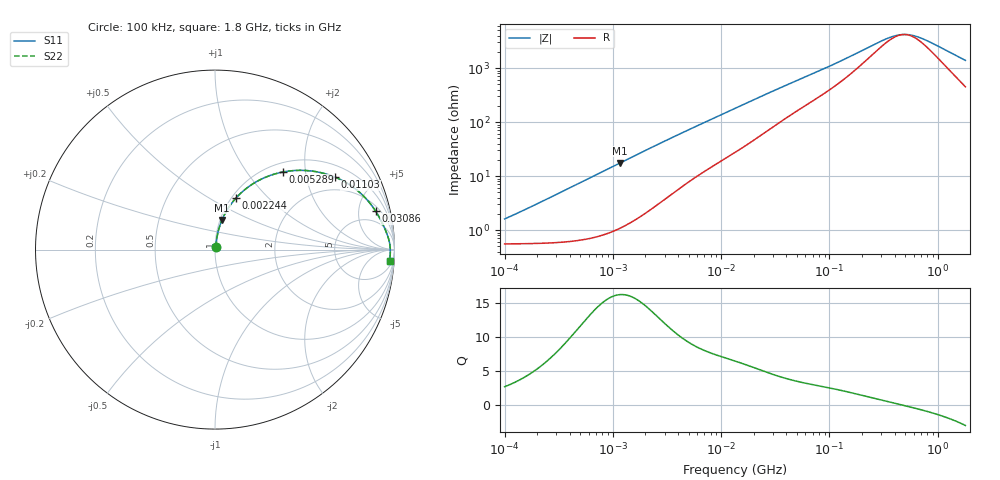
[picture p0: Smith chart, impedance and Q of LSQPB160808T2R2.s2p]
! LSQPB160808T2R2  S-PARAMETER MODEL  ( General Type )
! Model Generated by TAIYO YUDEN Corporation (http://www.ty-top.com)
! Version 4.0
! TAIYO YUDEN Control No. 100810NF18SB-HKC
! Copyright(c) 2007 TAIYO YUDEN CO.,LTD. All Rights Reserved.
! Product Description (link to TY-COMPAS)
! https://ds.yuden.co.jp/TYCOMPAS/or/detail?pn=LSQPB160808T2R2M&u=M
! Products Name : Inductors
! Characteristics :
!  Inductance : 2.2 uH , SRF(min) : 100 MHz , DC Resistance(max) : 0.715 Ohm
!  Rated Current : Saturation :550 mA , Temp Rise : 280 mA (40 degC)
!  Case Size : 1.6 x 0.8 / 0.063 x 0.031 [mm/inch] , Thickness : 0.8 / 0.031 [mm/inch]
!  (Conditions: Temperature = 25 degC , DC Bias Current/Voltage = 0A / 0V)
! External Node Assignments :
!  1  o---GGG---o  2
! GND o---------o GND
! Frequency Range : 0.1MHz  -  1800MHz  [ 402 STEP ]
# MHz S RI R 50
! Freq[MHz].  S11 Real  S11 Imag  S21 Real  S21 Imag  S12 Real  S12 Imag  S22 Real  S22 Imag
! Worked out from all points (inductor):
!   401 points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, 100 kHz to 1.8 GHz, reference 50 ohm
!   read as one part in series: L = 2.4 uH near 113 kHz
!   highest Q = 16.1 at 1.158 MHz (marker M1), where L = 2.39 uH
!   self-resonance near 485.7 MHz
!   S11 on the Smith chart (normalised r, x): 100 kHz: 1.01, +0.03; 2.244 MHz: 1.05, +0.67; 5.289 MHz: 1.17, +1.51; 11.03 MHz: 1.43, +2.96; 30.86 MHz: 2.68, +7.50; 1.8 GHz: 10, -26
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0.1  0.00573 0.0149  0.9943 -0.0149  0.9943 -0.0149  0.00573 0.0149
0.167264  0.00621 0.0249  0.9938 -0.0249  0.9938 -0.0249  0.00621 0.0249
0.516129  0.0124 0.0763  0.9876 -0.0763  0.9876 -0.0763  0.0124 0.0763
1.158292  0.0391 0.1654  0.9609 -0.1654  0.9609 -0.1654  0.0391 0.1654
1.632122  0.0693 0.2237  0.9307 -0.2237  0.9307 -0.2237  0.0693 0.2237
2.244135  0.1172 0.2875  0.8828 -0.2875  0.8828 -0.2875  0.1172 0.2875
2.66389  0.1535 0.3234  0.8465 -0.3234  0.8465 -0.3234  0.1535 0.3234
3.662795  0.2432 0.3851  0.7568 -0.3851  0.7568 -0.3851  0.2432 0.3851
5.289144  0.378 0.4324  0.622 -0.4324  0.622 -0.4324  0.378 0.4324
7.637621  0.528 0.439  0.472 -0.439  0.472 -0.439  0.528 0.439
11.02886  0.6686 0.4039  0.3314 -0.4039  0.3314 -0.4039  0.6686 0.4039
13.41641  0.7324 0.3722  0.2676 -0.3722  0.2676 -0.3722  0.7324 0.3722
19.85396  0.8295 0.2965  0.1705 -0.2965  0.1705 -0.2965  0.8295 0.2965
30.85563  0.8945 0.2149  0.1055 -0.2149  0.1055 -0.2149  0.8945 0.2149
69.24595  0.9484 0.1113  0.0516 -0.1113  0.0516 -0.1113  0.9484 0.1113
144.3909  0.9685 0.0551  0.0315 -0.0551  0.0315 -0.0551  0.9685 0.0551
357.3983  0.9761 0.0117  0.0239 -0.0117  0.0239 -0.0117  0.9761 0.0117
413.9822  0.9764 0.00604  0.0236 -0.00604  0.0236 -0.00604  0.9764 0.00604
479.5244  0.9767 0.000484  0.0233 -0.000484  0.0233 -0.000484  0.9767 0.000484
627.8136  0.9768 -0.0098  0.0232 0.0098  0.0232 0.0098  0.9768 -0.0098
842.3428  0.9766 -0.0219  0.0234 0.0219  0.0234 0.0219  0.9766 -0.0219
1800  0.9729 -0.0648  0.0271 0.0648  0.0271 0.0648  0.9729 -0.0648
